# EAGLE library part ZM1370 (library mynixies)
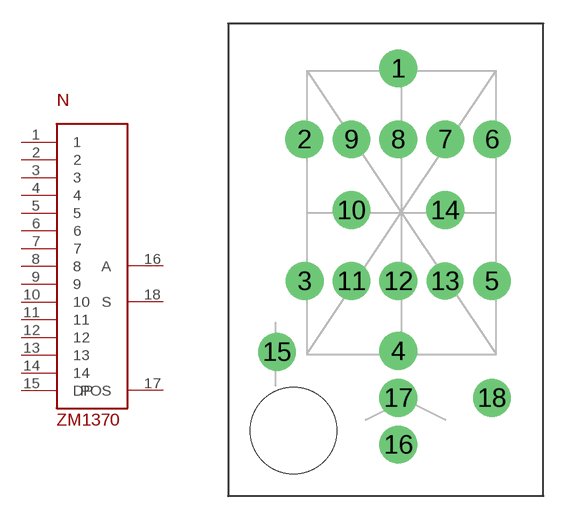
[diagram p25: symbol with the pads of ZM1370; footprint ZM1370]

Designator prefix N

## ZM1370  [ZM1370]
1  1  pas
2  2  pas
3  3  pas
4  4  pas
5  5  pas
6  6  pas
7  7  pas
8  8  pas
9  9  pas
10  10  pas
11  11  pas
12  12  pas
13  13  pas
14  14  pas
15  DP  pas
16  A  pas
17  POS  pas
18  S  pas

## Footprint ZM1370 (pad centres in mm)
drill 1.6: 1 0.8,12.15; 2 -5.17,7.65; 3 -5.14,-1.35; 4 0.8,-5.8; 5 6.74,-1.35; 6 6.74,7.65; 7 3.77,7.65; 8 0.8,7.65; 9 -2.17,7.65; 10 -2.17,3.15; 11 -2.17,-1.35; 12 0.8,-1.35; 14 3.77,3.15; 15 -6.9,-5.85; 16 0.8,-11.74; 17 0.8,-8.77; 18 6.74,-8.77
drill 1.55: 13 3.77,-1.35
hole 5.5 at -5.86,-10.85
